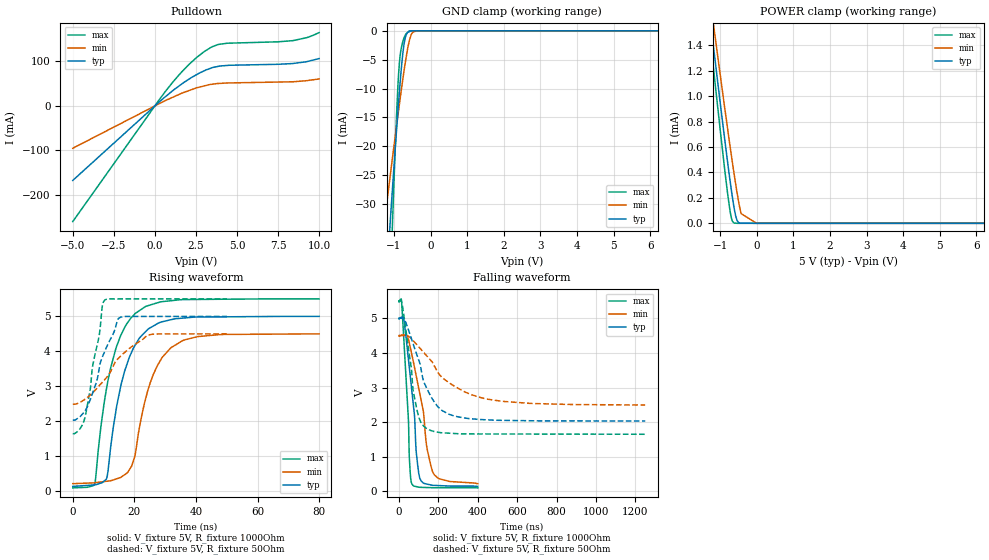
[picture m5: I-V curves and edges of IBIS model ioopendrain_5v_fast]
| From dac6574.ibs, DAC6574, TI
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|   ioopendrain_5v_fast Model
[Model]   ioopendrain_5v_fast
Model_type   I/O_open_drain
Polarity   Non-Inverting
Enable   Active-Low
Vinl = 1.5
Vinh = 3.5
Vmeas = 2.5
Vref = 5.0
Cref = 400pF
Rref = 1000
|   typ   min   max
|   (nom PVT)   (Fast PVT)   (slow PVT)
|Average
C_comp   5.061e-12   5.040e-12   5.094e-12
|ON state : BUFFER OUTPUT TURNED LOW
|C_comp   6.129e-11   2.855e-11   1.162e-10
|OFF state: BUFFER in HIGH IMPEDANCE
|C_comp   5.061e-12   5.040e-12   5.094e-12
| Where nom  PVT is Nominal Process, 5V, 25C
|   Fast PVT is Strong Process,  5.5V, -40C
|   Slow PVT is Weak Process,   4.5V, 105C
[Model spec]
|   typ   min   max
Vinl   1.5   1.35   1.65
Vinh   3.5   3.15   3.85
[Voltage Range]   5   4.5   5.5
|Ambient Temperature   25   105   -40
|Junction Temperature
[Temperature Range]   25   105   -40
[Pullup Reference]   5   4.5   5.5
[Pulldown Reference]   0   0   0
[Power Clamp Reference]   5   4.5   5.5
[GND Clamp Reference]   0   0   0
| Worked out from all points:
|   slope of the pulldown table from 0 to 0.75 V, typ, clamps not added: 31.1 ohm
|   GND clamp passes 1 mA (typ) near -0.68 V on its own axis
|   POWER clamp passes 1 mA (typ) near -1.02 V on its own axis
|   falling waveform, V_fixture 5V, R_fixture 1000Ohm: 20-80 % time 43.9ns typ, 72ns min, 27.1ns max; typ from 5 V to 0.145 V
|   rising waveform, V_fixture 5V, R_fixture 1000Ohm: 20-80 % time 7.25ns typ, 7.51ns min, 7.14ns max; typ from 0.145 V to 5 V
|   falling waveform, V_fixture 5V, R_fixture 50Ohm: 20-80 % time 111ns typ, 214ns min, 55.6ns max; typ from 5 V to 2.03 V
|   rising waveform, V_fixture 5V, R_fixture 50Ohm: 20-80 % time 6.86ns typ, 11.3ns min, 4.32ns max; typ from 2.03 V to 5 V
[Pulldown]
|   Voltage   I(typ)   I(min)   I(max)
-5V       -167.6mA   -95.21mA   -260.1mA
632mV     20.56mA    11.88mA    32.24mA
1.567V    47.51mA    27.48mA    73.88mA
2.073V    60.23mA    34.53mA    93.27mA
3.03V     79.48mA    45.34mA    123mA
3.475V    85.81mA    48.85mA    133mA
3.866V    89.13mA    50.56mA    138.4mA
4.41V     91.14mA    51.64mA    141.1mA
7.49V     93.71mA    53.75mA    144.3mA
8.398V    95.44mA    54.36mA    146.9mA
9.239V    99.6mA     56.83mA    153.6mA
10V       106.6mA    60.8mA     165.1mA
[GND Clamp]
|   Voltage   I(typ)   I(min)   I(max)
-5V       -412.1mA   -229.4mA   -786.8mA
-1.266V   -48.89mA   -33.49mA   -75.73mA
-1.101V   -33mA      -25.04mA   -44.62mA
-1.04V    -27.31mA   -21.99mA   -33.44mA
-924.5mV  -16.82mA   -16.27mA   -14.04mA
-886mV    -13.47mA   -14.41mA   -8.932mA
-847.5mV  -10.29mA   -12.56mA   -5.324mA
-725mV    -2.321mA   -6.967mA   -1.233mA
-581mV    0A         -1.729mA   -153.9uA
-495.5mV  0A         -326.8uA   0A
-324.5mV  0A         0A         0A
10V       0A         0A         0A
[POWER Clamp]
|   Voltage   I(typ)   I(min)   I(max)
-5V       10.92mA    10.1mA     11.74mA
-1.335V   1.762mA    1.9mA      1.632mA
-1.265V   1.591mA    1.747mA    1.443mA
-1.238V   1.526mA    1.688mA    1.371mA
-1.15V    1.313mA    1.498mA    1.136mA
-748.5mV  378.2uA    647.3uA    135.5uA
-688mV    251.5uA    526.5uA    38.06uA
-622mV    128.1uA    396.8uA    2.687uA
-535mV    22.14uA    238.1uA    65.67nA
-428mV    1.278uA    76.93uA    28.57nA
-5mV      0A         0A         0A
10V       0A         0A         0A
[Ramp]
R_load = 1000
|   typ   min   max
dV/dt_r   2.91312/7.22321e-09   2.56641/7.46433e-09   3.2383/7.13116e-09
dV/dt_f   2.91312/4.38564e-08   2.56634/7.17932e-08   3.2383/2.70617e-08
[Falling Waveform]
V_fixture = 5V
V_fixture_min = 4.5V
V_fixture_max = 5.5V
R_fixture = 1000Ohm
|   Time   V(typ)   V(min)   V(max)
0s        5V         4.5V       5.5V
13.91ns   5.029V     4.514V     5.443V
48.4ns    3.808V     4.383V     2.041V
53.53ns   3.537V     4.265V     902.7mV
66.19ns   2.869V     3.932V     209.5mV
79.54ns   2.153V     3.565V     149mV
87.59ns   1.149V     3.337V     139.1mV
105.3ns   391.4mV    2.837V     118.7mV
171.9ns   175.9mV    557.7mV    107.2mV
400ns     144.8mV    222.8mV    102.8mV
[Rising Waveform]
V_fixture = 5V
V_fixture_min = 4.5V
V_fixture_max = 5.5V
R_fixture = 1000Ohm
|   Time   V(typ)   V(min)   V(max)
0s        144.8mV    222.6mV    102.8mV
7.151ns   186.6mV    249.1mV    208.9mV
10.96ns   364.5mV    290.9mV    2.937V
15.62ns   3.024V     403.3mV    4.46V
20.25ns   4.176V     1.048V     5.079V
22.15ns   4.429V     2.063V     5.194V
25.23ns   4.678V     3.123V     5.327V
31.85ns   4.904V     4.103V     5.447V
40.57ns   4.981V     4.422V     5.484V
80ns      5V         4.5V       5.5V
[Falling Waveform]
V_fixture = 5V
V_fixture_min = 4.5V
V_fixture_max = 5.5V
R_fixture = 50Ohm
|   Time   V(typ)   V(min)   V(max)
0s        5V         4.5V       5.5V
17.42ns   4.998V     4.499V     5.374V
63.83ns   4.401V     4.407V     3.527V
72.07ns   4.261V     4.355V     2.92V
90.41ns   3.957V     4.238V     2.386V
110.6ns   3.583V     4.109V     2.005V
145.3ns   2.931V     3.888V     1.801V
251.1ns   2.236V     3.152V     1.682V
434.4ns   2.07V      2.682V     1.659V
1.25us    2.033V     2.494V     1.65V
[Rising Waveform]
V_fixture = 5V
V_fixture_min = 4.5V
V_fixture_max = 5.5V
R_fixture = 50Ohm
|   Time   V(typ)   V(min)   V(max)
0s        2.033V     2.492V     1.65V
3.947ns   2.297V     2.63V      2.11V
5.663ns   2.616V     2.751V     2.907V
6.435ns   2.807V     2.813V     3.572V
8.599ns   3.52V      3.021V     4.465V
9.654ns   3.846V     3.125V     5.321V
10.35ns   3.995V     3.193V     5.462V
15.5ns    4.976V     3.861V     5.498V
24.28ns   4.998V     4.463V     5.498V
50ns      5V         4.5V       5.5V
